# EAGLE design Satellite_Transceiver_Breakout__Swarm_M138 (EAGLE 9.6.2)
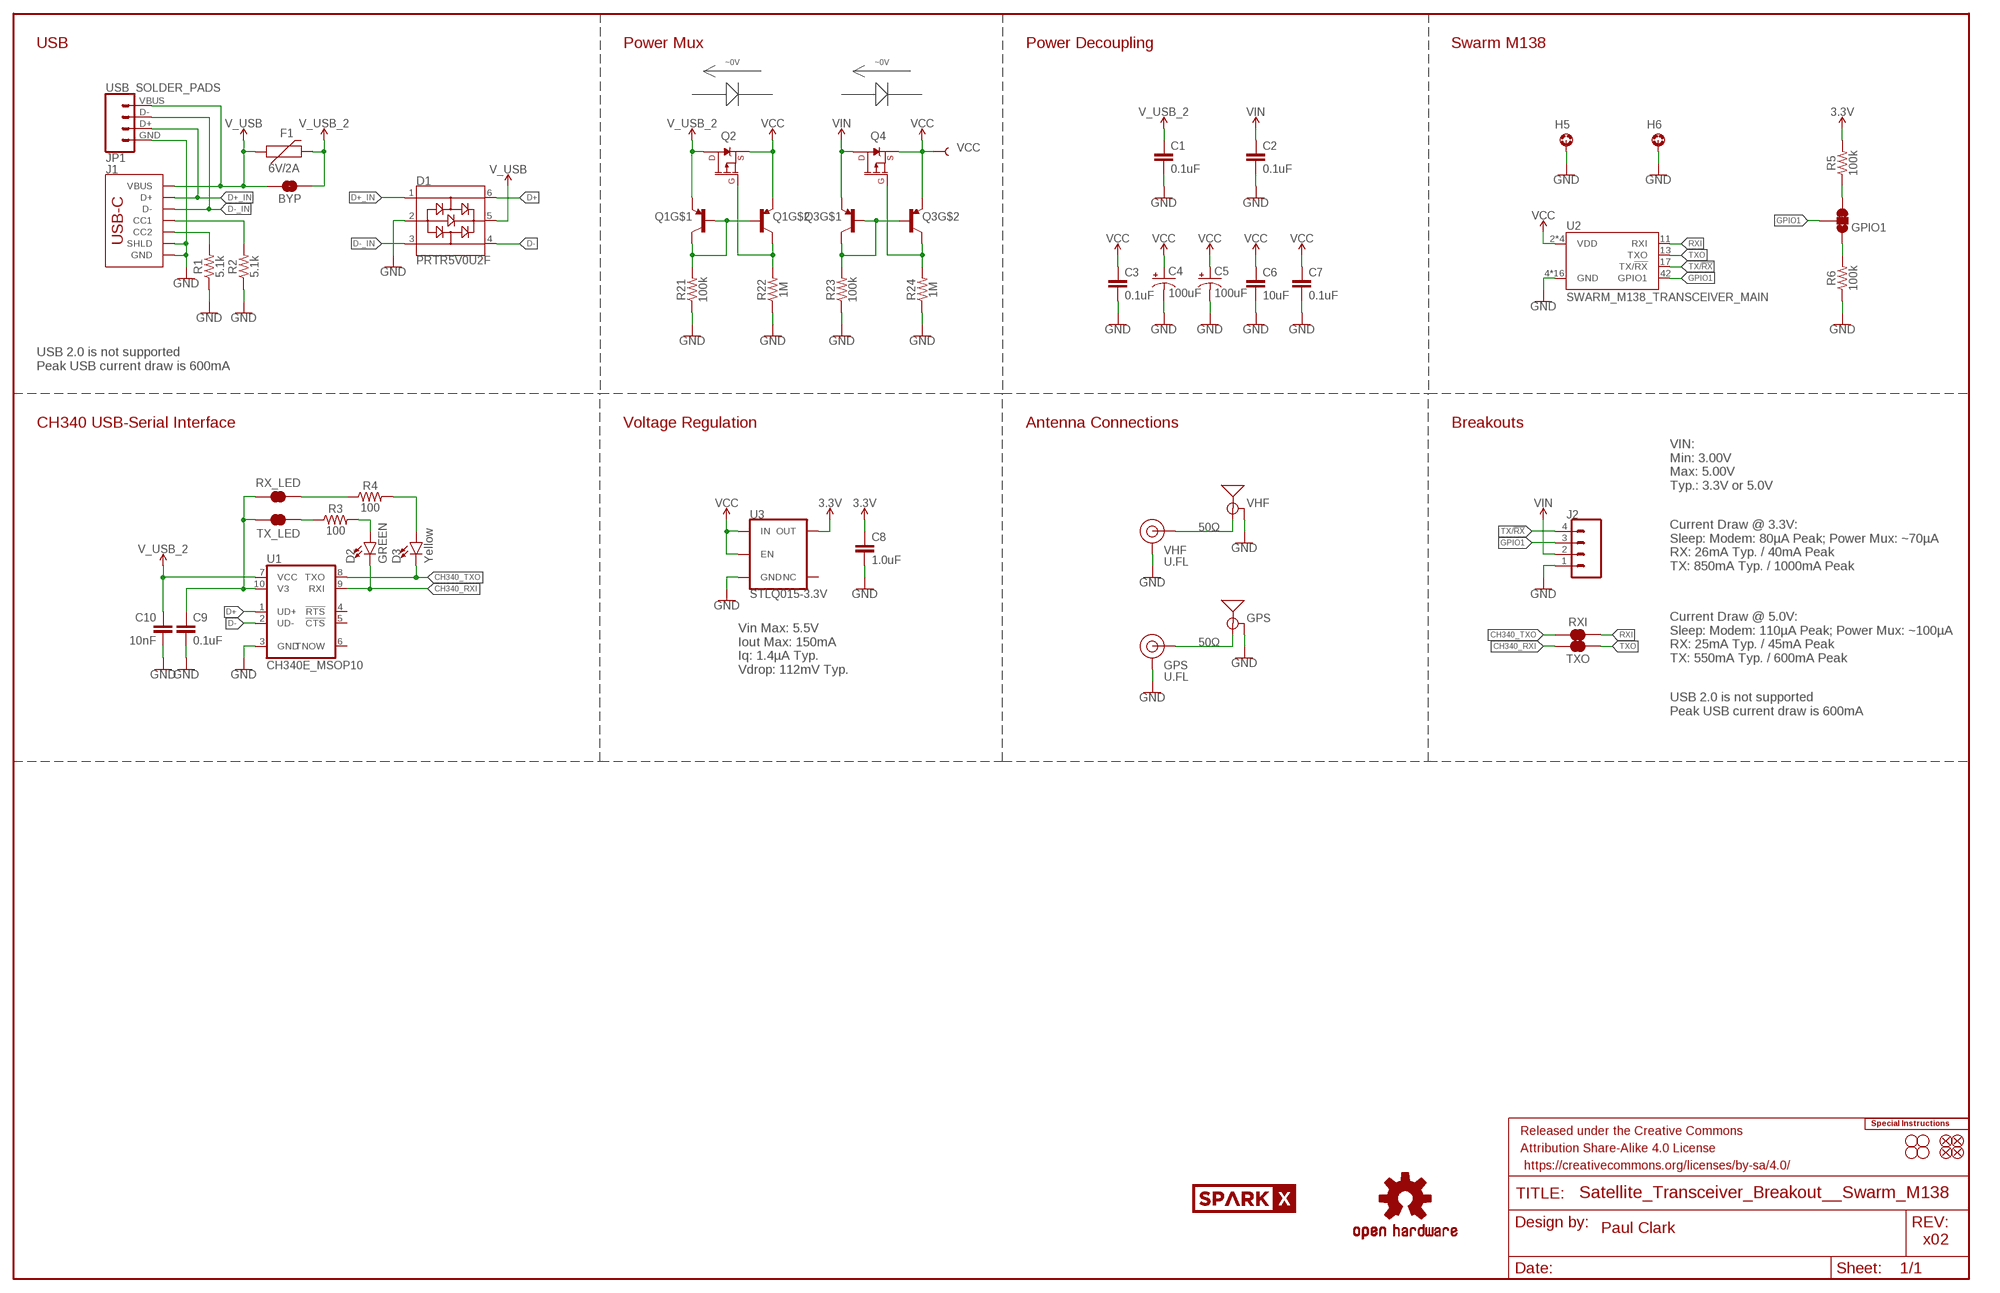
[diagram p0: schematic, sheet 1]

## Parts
BYP  JUMPER-SMT_2_NO_SILK  [SMT-JUMPER_2_NO_SILK]
C1  0.1uF  0.1UF-0603-25V-5%  [0603]
C2  0.1uF  0.1UF-0603-25V-5%  [0603]
C3  0.1uF  0.1UF-0603-25V-5%  [0603]
C4  100uF  100UF-POLAR-25V-20%(ELEC)  [PANASONIC_D]
C5  100uF  100UF-POLAR-25V-20%(ELEC)  [PANASONIC_D]
C6  10uF  10UF-0603-6.3V-20%  [0603]
C7  0.1uF  0.1UF-0603-25V-5%  [0603]
C8  1.0uF  1.0UF-0603-16V-10%-X7R  [0603]
C9  0.1uF  0.1UF-0603-25V-5%  [0603]
C10  10nF  10NF-0603-50V-10%  [0603]
D1  PRTR5V0U2F  [SOT886]
D2  GREEN  LED-GREEN0603  [LED-0603]
D3  Yellow  LED-YELLOW0603  [LED-0603]
E1  VHF  ANTENNA-SMA-GROUNDEDEDGE_SMA  [SMA-EDGE]
E2  GPS  ANTENNA-SMA-GROUNDEDEDGE_SMA  [SMA-EDGE]
F1  6V/2A  PPTC_6V2A  [1210]
FD1  FIDUCIAL1X2  [FIDUCIAL-1X2]
FD2  FIDUCIAL1X2  [FIDUCIAL-1X2]
FD3  FIDUCIAL1X2  [FIDUCIAL-1X2]
FD4  FIDUCIAL1X2  [FIDUCIAL-1X2]
FRAME1  FRAME-LEDGER  [CREATIVE_COMMONS]
GPIO1  JUMPER-SMT_3_1-NC_TRACE_SILK  [SMT-JUMPER_3_1-NC_TRACE_SILK]
GPS  U.FL  U.FL2PIN  [U.FL]
H1  STAND-OFF  [STAND-OFF]
H2  STAND-OFF  [STAND-OFF]
H3  STAND-OFF  [STAND-OFF]
H4  STAND-OFF  [STAND-OFF]
H5  STAND-OFF-REFLOW-M2.5_1.5MM_TALL  [STAND-OFF-REFLOW-M2.5]
H6  STAND-OFF-REFLOW-M2.5_1.5MM_TALL  [STAND-OFF-REFLOW-M2.5]
J1  USB_C_2-LAYER_PADS  [USB-C-16P-2LAYER-PADS]
J2  CONN_041X04_NO_SILK  [1X04_NO_SILK]
JP1  USB_SOLDER_PADS  [USB-SOLDER-PADS]
LOGO1  SPECIAL_INSTRUCTIONS-ORDERING  [ORDERING_INSTRUCTIONS]
LOGO2  OSHW-LOGOM  [OSHW-LOGO-M]
LOGO3  OSHW-LOGOM  [OSHW-LOGO-M]
Q1  TRANS_PNP_DUALSOT-363  [SOT363_PHILIPS]
Q2  20V/4.2A/52mΩ/1.4W  MOSFET_PCH-DMG2305UX-7  [SOT23-3]
Q3  TRANS_PNP_DUALSOT-363  [SOT363_PHILIPS]
Q4  20V/4.2A/52mΩ/1.4W  MOSFET_PCH-DMG2305UX-7  [SOT23-3]
R1  5.1k  5.1KOHM5.1KOHM-0603-1/10W-1%  [0603]
R2  5.1k  5.1KOHM5.1KOHM-0603-1/10W-1%  [0603]
R3  100  100OHM-0603-1/10W-1%  [0603]
R4  100  100OHM-0603-1/10W-1%  [0603]
R5  100k  100KOHM-0603-1/10W-1%  [0603]
R6  100k  100KOHM-0603-1/10W-1%  [0603]
R21  100k  100KOHM-0603-1/10W-1%  [0603]
R22  1M  1MOHM-0603-1/4W-5%  [0603]
R23  100k  100KOHM-0603-1/10W-1%  [0603]
R24  1M  1MOHM-0603-1/4W-5%  [0603]
RX_LED  JUMPER-SMT_2_NC_TRACE_SILK  [SMT-JUMPER_2_NC_TRACE_SILK]
RXI  JUMPER-COMBO_2_NC_TRACE  [COMBO-JUMPER_2_NC_TRACE]
TX_LED  JUMPER-SMT_2_NC_TRACE_SILK  [SMT-JUMPER_2_NC_TRACE_SILK]
TXO  JUMPER-COMBO_2_NC_TRACE  [COMBO-JUMPER_2_NC_TRACE]
U1  CH340E_MSOP10  [MSOP10]
U2  SWARM_M138_TRANSCEIVER_MAIN  [M.2-SWARM-M138-A]
U3  STLQ015-3.3V  [SOT23-5]
U$1  SPARKX-LOGO5  [SPARKX-LARGE]
U$2  SPARKX-LOGO5  [SPARKX-LARGE]
VCC  TEST-POINT3X5  [PAD.03X.05]
VHF  U.FL  U.FL2PIN  [U.FL]

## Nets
3.3V: C8.1 R5.2 U3.5(OUT)
CH340_RXI: D2.C TXO.2 TXO.4 U1.9(RXI)
CH340_TXO: D3.C RXI.1 RXI.3 U1.8(TXO)
D+: D1.6 U1.1(UD+)
D+_IN: D1.1 J1.A6(D+) J1.B6(D+) JP1.D+
D-: D1.4 U1.2(UD-)
D-_IN: D1.3 J1.A7(D-) J1.B7(D-) JP1.D-
GND: C1.2 C2.2 C3.2 C4.- C5.- C6.2 C7.2 C8.2 C9.2 C10.2 D1.2 E1.GND@0(GND) E1.GND@1(GND) E1.GND@2(GND) E1.GND@3(GND) E2.GND@0(GND) E2.GND@1(GND) E2.GND@2(GND) E2.GND@3(GND) GPS.1(GND) GPS.2(GND) H5.1 H6.1 J1.GND J1.GND2(GND) J1.SHLD1(SHLD) J1.SHLD2(SHLD) J1.SHLD3(SHLD) J1.SHLD4(SHLD) J2.1 JP1.GND R1.1 R2.1 R6.1 R21.1 R22.1 R23.1 R24.1 U1.3(GND) U2.4(GND) U2.9(GND) U2.15(GND) U2.18(GND) U2.21(GND) U2.26(GND) U2.27(GND) U2.29(GND) U2.34(GND) U2.35(GND) U2.37(GND) U2.40(GND) U2.43(GND) U2.50(GND) U2.A1(GND) U2.A2(GND) U3.2(GND) VHF.1(GND) VHF.2(GND)
GPIO1: GPIO1.2 J2.3 U2.42(GPIO1)
GPS: E2.SIG(SIGNAL) GPS.FEED(SIGNAL)
N$2: J1.B5(CC2) R1.2
N$3: J1.A5(CC1) R2.2
N$5: Q1.2(B) Q1.5(B) Q1.6(C) R21.2
N$6: C9.1 RX_LED.1 TX_LED.2 U1.10(V3)
N$7: R4.1 RX_LED.2
N$9: D2.A R3.2
N$10: D3.A R4.2
N$12: R3.1 TX_LED.1
N$13: Q1.3(C) Q2.1(G) R22.2
N$14: GPIO1.3 R5.1
N$15: Q3.2(B) Q3.5(B) Q3.6(C) R23.2
N$16: GPIO1.1 R6.2
N$28: Q3.3(C) Q4.1(G) R24.2
RXI: RXI.2 RXI.4 U2.11(RXI)
TX/!RX!: J2.4 U2.17(TX/!RX!)
TXO: TXO.1 TXO.3 U2.13(TXO)
V_USB: BYP.2 D1.5 F1.1 J1.VBUS1(VBUS) J1.VBUS2(VBUS) JP1.VBUS
V_USB_2: BYP.1 C1.1 C10.1 F1.2 Q1.1(E) Q2.3(D) U1.7(VCC)
VCC: C3.1 C4.+ C5.+ C6.1 C7.1 Q1.4(E) Q2.2(S) Q3.4(E) Q4.2(S) U2.2(VDD) U2.39(VDD) U2.41(VDD) U2.52(VDD) U3.1(IN) U3.3(EN) VCC.1
VHF: E1.SIG(SIGNAL) VHF.FEED(SIGNAL)
VIN: C2.1 J2.2 Q3.1(E) Q4.3(D)
Unconnected: U1.4(!RTS) U1.5(!CTS) U1.6(TNOW) U3.4(NC)

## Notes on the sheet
- USB | Power Mux | Power Decoupling | Swarm M138
- ~0V | ~0V
- USB 2.0 is not supported
  Peak USB current draw is 600mA
- CH340 USB-Serial Interface | Voltage Regulation | Antenna Connections | Breakouts
- VIN:
  Min: 3.00V
  Max: 5.00V
  Typ.: 3.3V or 5.0V
- Current Draw @ 3.3V:
  Sleep: Modem: 80µA Peak; Power Mux: ~70µA
  RX: 26mA Typ. / 40mA Peak
  TX: 850mA Typ. / 1000mA Peak
- 50Ω
- Current Draw @ 5.0V:
  Sleep: Modem: 110µA Peak; Power Mux: ~100µA
  RX: 25mA Typ. / 45mA Peak
  TX: 550mA Typ. / 600mA Peak
- Vin Max: 5.5V
  Iout Max: 150mA
  Iq: 1.4µA Typ.
  Vdrop: 112mV Typ.
- 50Ω
- USB 2.0 is not supported
  Peak USB current draw is 600mA
- Paul Clark
- x02

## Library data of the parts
BYP = SparkFun-Jumpers:JUMPER-SMT_2_NO: Normally open jumper
C1-C3 C7 C9 = SparkFun-Capacitors:0.1UF: 0.1µF ceramic capacitors; PROD_ID: CAP-08604
C4 C5 = SparkFun-Capacitors:100UF-POLAR: 100µF polarized capacitors; PROD_ID: CAP-12547
C6 = SparkFun-Capacitors:10UF: 10.0µF ceramic capacitors; PROD_ID: CAP-11015
C8 = SparkFun-Capacitors:1.0UF: 1µF ceramic capacitors; PROD_ID: CAP-13930
C10 = SparkFun-Capacitors:10NF: 0.01uF/10nF/10,000pF ceramic capacitors; PROD_ID: CAP-00867
D1 = SparkFun-IC-Power:PRTR5V0U2: A small ESD protection device. Most commonly used on USB D+/D- signals to protect large, expensive, or especially sensitive USB enabled devices.; PROD_ID: DIO-14084
D2 = SparkFun-LED:LED-GREEN: Green SMD LED; PROD_ID: DIO-00821
D3 = SparkFun-LED:LED-YELLOW: Yellow SMD LED; PROD_ID: DIO-09003
E1 E2 = SparkFun-RF:ANTENNA-SMA-GROUNDED: SMA Antenna Connector w/ Ground; PROD_ID: CONN-08289
F1 = SparkFun-Fuses:PPTC: Resettable Fuse PPTC; PROD_ID: RES-14313
FD1-FD4 = SparkFun-Aesthetics:FIDUCIAL: Fiducial Alignment Points
FRAME1 = SparkFun-Aesthetics:FRAME-LEDGER: Schematic Frame - Ledger
GPIO1 = SparkFun-Jumpers:JUMPER-SMT_3_1-NC_TRACE: Normally closed trace jumper (1 of 2 connections) This jumper has a trace between two pads so it's normally closed (NC). The other connection is normally open (NO). Use a razor knife to open the connection. For best results follow the IPC guidelines for cutting traces: Cutout at least 0.063 mm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
GPS VHF = SparkFun-Connectors:U.FL2PIN: SMD Antenna Connector - U.FL; PROD_ID: CONN-09193; SF_ID: WRL-09144
H1-H4 = SparkFun-Hardware:STAND-OFF: Stand Off
H5 H6 = SparkFun-Hardware:STAND-OFF-REFLOW: Stand Off Reflow Compatible; PROD_ID: HW-16629
J1 = SparkFun-Connectors:USB_C: USB Type C 16Pin Connector Super Speed pins not available on the 16-pin purely SMD connector so this part is best for USB 2.0 implementations. D1 and D2 are tied together enabling D+/- no matter which way the cable is plugged into the connector. The two channel configuration pins (CC1/2) are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; PROD_ID: CONN-14122
J2 = SparkFun-Connectors:CONN_04: Multi connection point. Often used as Generic Header-pin footprint for 0.1 inch spaced/style header connections On any of the 0.1 inch spaced packages, you can populate with these: Break Away Headers - Straight (PRT-00116) Break Away Male Headers - Right Angle (PRT-00553) Female Headers (PRT-00115)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; PROD_ID: CONN-09696
JP1 = SparkFun-Connectors:USB_SOLDER_PADS: Solder pad access to USB pins. Helpful to expose on PCBs so user can attach external USB connector if necessary.
LOGO1 = SparkFun-Aesthetics:SPECIAL_INSTRUCTIONS: Special Ordering/Production Instructions Alert
LOGO2 LOGO3 = SparkFun-Aesthetics:OSHW-LOGO: Open-Source Hardware (OSHW) Logo
Q1 Q3 = SparkFun-DiscreteSemi:TRANS_PNP_DUAL: Dual PNP Transistors in Single Package The BCM857BS puts two PNP transistors in a single package. Bipolar (BJT) Transistor Array 2 PNP (Dual) 45V 100mA 100MHz 200mW Surface Mount SOT-363 Datasheet SparkFun Products: SparkFun Pi Servo HAT V2; PROD_ID: TRANS-14386
Q2 Q4 = SparkFun-DiscreteSemi:MOSFET_PCH: P-channel MOSFETs Voltage controlled devices that allow control of high current outputs. SparkFun Products: SparkFun ESP32 Thing SparkFun ESP8266 Thing SparkFun Pi Servo HAT V2 DMG2305UX-7 (20V/4.2A/SOT23-3); PROD_ID: TRANS-14388
R1 R2 = SparkFun-Resistors:5.1KOHM; PROD_ID: RES-12083
R3 R4 = SparkFun-Resistors:100OHM: 100Ω resistor; PROD_ID: RES-07863
R5 R6 R21 R23 = SparkFun-Resistors:100KOHM: 100kΩ resistor; PROD_ID: RES-07828
R22 R24 = SparkFun-Resistors:1MOHM: 1MΩ resistor; PROD_ID: RES-07868
RX_LED TX_LED = SparkFun-Jumpers:JUMPER-SMT_2_NC_TRACE: Normally closed trace jumper
RXI TXO = SparkFun-Jumpers:JUMPER-COMBO_2_NC_TRACE
U1 = SparkFun-IC-Comms:CH340E; PROD_ID: IC-14135
U2 = Swarm:SWARM_M138_TRANSCEIVER: Swarm M138 Modem Description: A satellite transceiver based on the mPCIe standard.; PROD_ID: CONN-16558
U3 = SparkFun-IC-Power:STLQ015: STLQ015 - 150mA CMOS LDO Regulator w/ Enable 1.4uA quiescent; PROD_ID: IC-15779
U$1 U$2 = SparkX:SPARKX-LOGO
VCC = SparkFun-Connectors:TEST-POINT: SparkFun Test Points

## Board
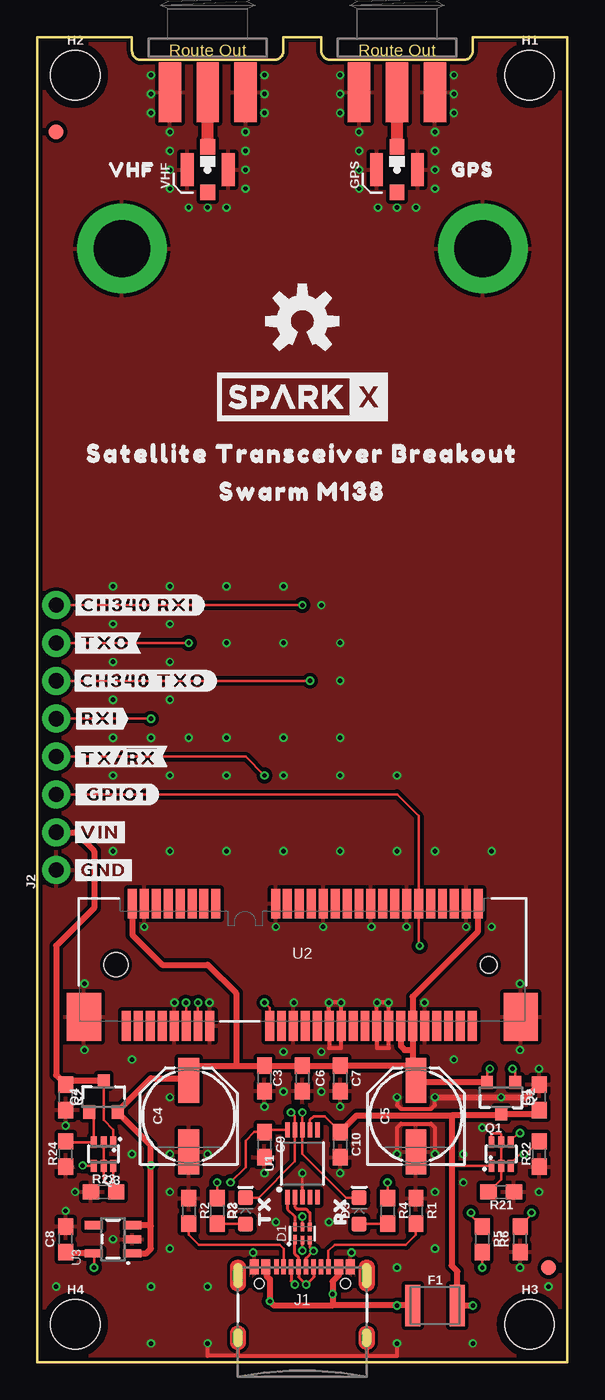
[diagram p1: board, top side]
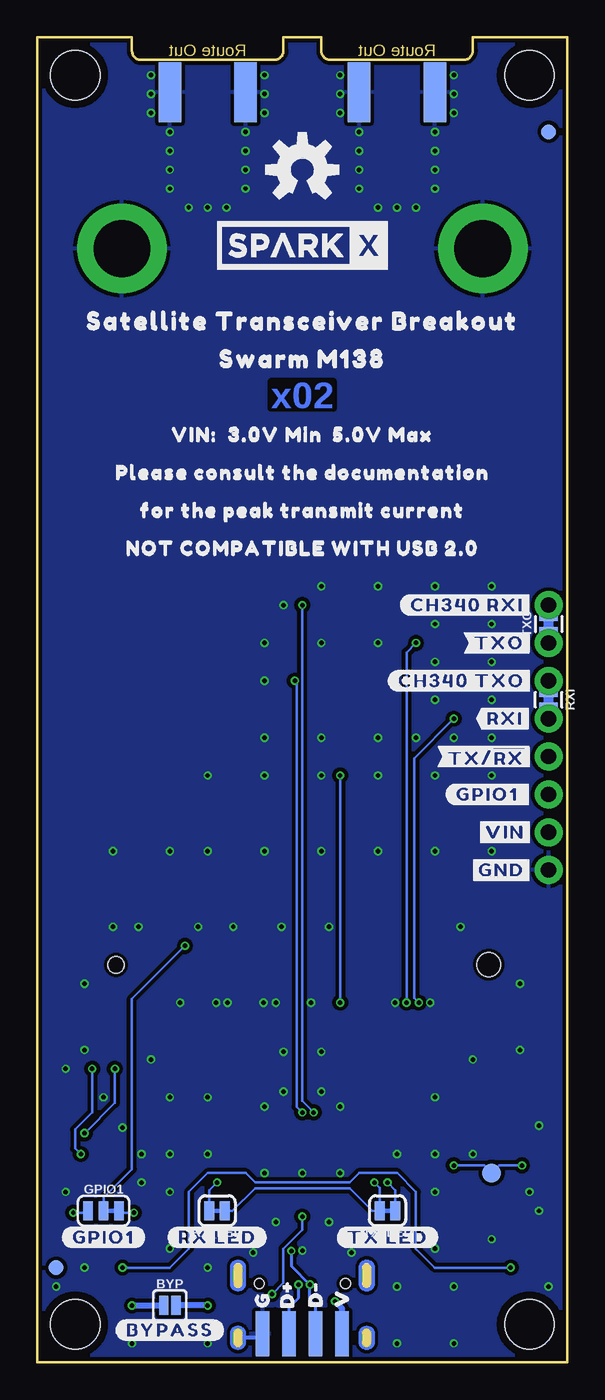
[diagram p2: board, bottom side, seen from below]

Size 35.56 x 88.9 mm. Coordinates in mm from the lower left corner, seen from the top.
Outline: 0,0 35.56,0 35.56,88.9 29.21,88.9 29.21,88.01 arc-90 28.57,87.38 19.68,87.38 arc-90 19.05,88.01 19.05,88.9 16.51,88.9 16.51,88.01 arc-90 15.88,87.38 6.99,87.38 arc-90 6.35,88.01 6.35,88.9 0,88.9 0,0
Copper layers (1*16): Top 0.035mm / dielectric 1.5mm / Bottom 0.035mm
Design rules "SparkFun-2-Layer-Minimum-JLCPCB": minimum track width 5mil, minimum drill 0.3mm, track to track 5mil, track to pad 5mil, pad to pad 5mil, via to via 5mil, smd to smd 5mil, copper to edge 7mil, drill to drill 7mil, minimum pad ring 5mil, minimum via ring 5mil, stop-mask expansion 2.5mil, vias tented up to drill 25mil, thermal gap 10mil
tRestrict: area 10.7,79.1 to 12.2,80.9; area 23.4,79.1 to 24.9,80.9; 4 lines
bRestrict: 3 lines

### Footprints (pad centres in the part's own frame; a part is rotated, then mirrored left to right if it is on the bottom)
SMT-JUMPER_2_NO_SILK = smd 0.635 x 1.27: 1 -0.406,0; 2 0.406,0
0603 = smd 1.1 x 1: 1 -0.85,0; 2 0.85,0
PANASONIC_D = smd 3 x 1.4: + 2.4,0; - -2.4,0
SOT886 = smd 0.61 x 0.25: 1 -0.405,0.5 | smd 0.56 x 0.25: 2 -0.43,0; 3 -0.43,-0.5; 4 0.43,-0.5; 5 0.43,0; 6 0.43,0.5
LED-0603 = smd 1 x 1: A -0.877,0; C 0.877,0
SMA-EDGE = smd 1.5 x 4: GND@0 -2.54,0; GND@1 2.54,0; SIG 0,0 | smd 1.5 x 4 bottom: GND@2 -2.54,0; GND@3 2.54,0
1210 = smd 1 x 2.8: 1 -1.5,0; 2 1.5,0
FIDUCIAL-1X2 = smd 1 x 1: 1 0,0
SMT-JUMPER_3_1-NC_TRACE_SILK = smd 0.66 x 1.27: 1 -1.041,0; 2 0,0; 3 1.041,0
U.FL = smd 2.2 x 0.85: 1 0,1.375; 2 0,-1.375 | smd 1.05 x 1: FEED 1.525,0; NC -1.525,0
STAND-OFF = hole 3.302: 0,0
STAND-OFF-REFLOW-M2.5 = drill 3.8 pad 6: 1 0,0
USB-C-16P-2LAYER-PADS = smd 0.3 x 1: A5 -1.25,-0.34; A6 -0.25,-0.34; A7 0.25,-0.34; A8 1.25,-0.34; B5 1.75,-0.34; B6 0.75,-0.34; B7 -0.75,-0.34; B8 -1.75,-0.34 | smd 0.6 x 1: GND -3.225,-0.34; GND2 3.225,-0.34; VBUS1 -2.45,-0.34; VBUS2 2.45,-0.34 | drill 0.4 pad 0.6 long: SHLD1 -4.318,-0.915; SHLD2 4.318,-0.915; SHLD3 -4.318,-5.095; SHLD4 4.318,-5.095 | hole 0.65: -2.89,-1.445; 2.89,-1.445
1X04_NO_SILK = drill 1.016 pad 1.88: 1 0,0; 2 2.54,0; 3 5.08,0; 4 7.62,0
USB-SOLDER-PADS = smd 3 x 0.9: D+ 0,-0.889; D- 0,0.889; GND 0,-2.667; VBUS 0,2.667
SOT363_PHILIPS = smd 0.4 x 0.8: 1 -0.65,-0.8; 2 0,-0.8; 3 0.65,-0.8; 4 0.65,0.8; 5 0,0.8; 6 -0.65,0.8
SOT23-3 = smd 0.8 x 0.9: 1 -0.95,-1; 2 0.95,-1; 3 0,1.1
SMT-JUMPER_2_NC_TRACE_SILK = smd 0.66 x 1.27: 1 -0.521,0; 2 0.521,0
COMBO-JUMPER_2_NC_TRACE = smd 0.635 x 1.27: 1 -0.508,0; 2 0.508,0 | drill 1.016 pad 1.88: 3 -1.27,0; 4 1.27,0
MSOP10 = smd 1 x 0.3: 1 -2.25,1; 2 -2.25,0.5; 3 -2.25,0; 4 -2.25,-0.5; 5 -2.25,-1; 6 2.25,-1; 7 2.25,-0.5; 8 2.25,0; 9 2.25,0.5; 10 2.25,1
M.2-SWARM-M138-A = smd 0.6 x 2: 1 -11.8,-4.1; 2 -11.4,4.1; 3 -11,-4.1; 4 -10.6,4.1; 5 -10.2,-4.1; 6 -9.8,4.1; 7 -9.4,-4.1; 8 -9,4.1; 9 -8.6,-4.1; 10 -8.2,4.1; 11 -7.8,-4.1; 12 -7.4,4.1; 13 -7,-4.1; 14 -6.6,4.1; 15 -6.2,-4.1; 16 -5.8,4.1; 17 -2.2,-4.1; 18 -1.8,4.1; 19 -1.4,-4.1; 20 -1,4.1; 21 -0.6,-4.1; 22 -0.2,4.1; 23 0.2,-4.1; 24 0.6,4.1; 25 1,-4.1; 26 1.4,4.1; 27 1.8,-4.1; 28 2.2,4.1; 29 2.6,-4.1; 30 3,4.1; 31 3.4,-4.1; 32 3.8,4.1; 33 4.2,-4.1; 34 4.6,4.1; 35 5,-4.1; 36 5.4,4.1; 37 5.8,-4.1; 38 6.2,4.1; 39 6.6,-4.1; 40 7,4.1; 41 7.4,-4.1; 42 7.8,4.1; 43 8.2,-4.1; 44 8.6,4.1; 45 9,-4.1; 46 9.4,4.1; 47 9.8,-4.1; 48 10.2,4.1; 49 10.6,-4.1; 50 11,4.1; 51 11.4,-4.1; 52 11.8,4.1 | smd 2.3 x 3.2: A1 -14.65,-3.5; A2 14.65,-3.5 | hole 1.1: 12.5,0 | hole 1.6: -12.5,0
SOT23-5 = smd 0.55 x 1.2: 1 -0.95,-1.3; 2 0,-1.3; 3 0.95,-1.3; 4 0.95,1.3; 5 -0.95,1.3
PAD.03X.05 = smd 1.27 x 1.27: 1 0,0

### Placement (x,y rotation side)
BYP  26.67,3.81 0 bottom
C1  33.66,17.78 90 top
C2  1.91,17.78 270 top
C3  15.24,19.05 270 top
C4  10.16,16.51 90 top
C5  25.4,16.51 90 top
C6  17.78,19.05 270 top
C7  20.32,19.05 270 top
C8  1.91,8.26 90 top
C9  15.24,14.61 270 top
C10  20.32,14.61 270 top
D1  17.78,8.64 90 top
D2  13.97,10.16 90 top
D3  21.59,10.16 90 top
E1  11.43,85.22 0 top
E2  24.13,85.22 0 top
F1  26.67,3.81 0 top
FD1  34.29,6.35 0 top
FD2  34.29,6.35 0 bottom
FD3  1.27,82.55 0 top
FD4  1.27,82.55 0 bottom
FRAME1  not placed on the board
GPIO1  31.11,10.16 0 bottom
GPS  24.13,80.01 90 top
H1  33.02,86.36 0 top
H2  2.54,86.36 0 top
H3  33.02,2.54 0 top
H4  2.54,2.54 0 top
H5  5.68,74.72 0 top
H6  29.88,74.72 0 top
J1  17.78,6.73 0 top
J2  1.27,33.02 90 top
JP1  17.78,1.91 270 bottom
LOGO1  not placed on the board
LOGO2  17.78,69.85 0 top
LOGO3  17.78,80.01 0 bottom
Q1  31.11,13.97 0 top
Q2  31.11,17.78 180 top
Q3  4.45,13.97 180 top
Q4  4.45,17.78 0 top
R1  25.4,10.16 270 top
R2  10.16,10.16 270 top
R3  12.06,10.16 270 top
R4  23.5,10.16 270 top
R5  29.84,8.26 270 top
R6  32.38,8.26 90 top
R21  31.11,11.43 180 top
R22  33.66,13.97 90 top
R23  4.45,11.43 0 top
R24  1.91,13.97 90 top
RX_LED  23.5,10.16 180 bottom
RXI  1.27,44.45 270 bottom
TX_LED  12.06,10.16 180 bottom
TXO  1.27,49.53 90 bottom
U1  17.78,13.34 90 top
U2  17.78,26.67 0 top
U3  5.08,8.26 90 top
U$1  17.78,74.93 0 bottom
U$2  17.78,64.77 0 top
U$3  [VHF0]  6.35,80.01 0 top
U$4  [GPS0]  29.21,80.01 0 top
U$5  [VIN#__3#0V_MIN__5#0V_MAX0]  17.78,62.23 0 bottom
U$6  [PLEASE_CONSULT_THE_DOCUMENTATION0]  17.78,59.69 0 bottom
U$7  [#CH340_RXI#0]  6.73,50.8 0 top
U$8  [#CH340_RXI#341]  6.73,50.8 0 bottom
U$9  [#TXO#341]  4.57,48.26 0 top
U$10  [#TXO#342]  4.57,48.26 0 bottom
U$11  [#CH340_TXO#0]  7.11,45.72 0 top
U$12  [#CH340_TXO#341]  7.11,45.72 0 bottom
U$13  [#RXI#0]  4.19,43.18 0 bottom
U$14  [#RXI#1]  4.19,43.18 0 top
U$15  [#TX##RX##1]  5.46,40.64 0 bottom
U$16  [#TX##RX##0]  5.46,40.64 0 top
U$17  [#GPIO1_#2]  5.21,38.1 0 bottom
U$18  [V0]  15.11,4.32 90 bottom
U$19  [#GPIO1#0]  31.11,8.38 0 bottom
U$20  [#_GPIO1#2]  5.21,38.1 0 top
U$21  [#VIN#0]  4.19,35.56 0 top
U$22  [#VIN#0]  4.19,35.56 0 bottom
U$23  [#GND#0]  4.45,33.02 0 top
U$24  [#GND#0]  4.45,33.02 0 bottom
U$25  [TX0]  15.24,10.16 90 top
U$26  [RX0]  20.32,10.16 90 top
U$27  [#TX_LED#0]  12.06,8.38 0 bottom
U$28  [#RX_LED#0]  23.5,8.38 0 bottom
U$29  [#BYPASS#0]  26.67,2.16 0 bottom
U$30  [G3]  20.45,4.19 90 bottom
U$31  [FOR_THE_PEAK_TRANSMIT_CURRENT1]  17.78,57.15 0 bottom
U$32  [NOT_COMPATIBLE_WITH_USB_2#02]  17.78,54.61 0 bottom
U$34  [SATELLITE_TRANSCEIVER_BREAKOUT0]  17.78,60.96 0 top
U$36  [D#2]  18.8,4.57 90 bottom
U$37  [D#1]  16.89,4.57 90 bottom
U$39  [SATELLITE_TRANSCEIVER_BREAKOUT0]  17.78,69.85 0 bottom
U$40  [SWARM_M1381]  17.78,58.42 0 top
U$41  [SWARM_M1381]  17.78,67.31 0 bottom
VCC  5.08,12.7 0 bottom
VHF  11.43,80.01 90 top

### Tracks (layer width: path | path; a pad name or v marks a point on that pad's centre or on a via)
3.3V  (via drill 0.3)
  Top 0.152: U3.5 3.81,7.28 v3.81,6.35 | v29.84,6.35 R5.2
  Top 0.406: U3.5 2,7.3 C8.1
  Bottom 0.152: v29.84,6.35 26.67,6.35 25.4,7.62 25.4,11.43 24.13,12.7 21.59,12.7 20.95,12.06 14.61,12.06 13.97,12.7 11.43,12.7 10.16,11.43 10.16,7.62 8.89,6.35 v3.81,6.35
CH340_RXI  (via drill 0.3)
  Top 0.152: D2.C 14.85,11.04 17.28,13.47 U1.9 17.28,16.5 v17.02,16.76 | TXO.4 v17.78,50.8
  Bottom 0.152: TXO.4 TXO.2 | v17.02,16.76 17.78,17.53 v17.78,50.8
CH340_TXO  (via drill 0.3)
  Top 0.152: D3.C 20.71,11.04 17.78,13.97 U1.8 v17.78,16.76 | v18.29,45.72 RXI.3
  Bottom 0.152: RXI.3 RXI.1 | v17.78,16.76 18.16,17.14 18.16,45.59 v18.29,45.72
D+
  Top 0.203: U1.1 16.78,10.27 17.27,9.78 D1.6
D+_IN  (via drill 0.3)
  Top 0.203: D1.1 17.27,7.29 17.53,7.03 J1.A6 17.53,5.71 v18.03,5.21 18.53,5.7 J1.B6
  Bottom 0.203: v18.03,5.21 18.03,4.32 18.67,3.68 JP1.D+
D-
  Top 0.203: U1.2 17.28,10.41 17.4,10.29 18.03,10.29 18.29,10.03 D1.4
D-_IN  (via drill 0.3)
  Top 0.203: J1.A7 18.03,6.98 v18.52,7.47 18.28,7.71 D1.3 | J1.B7 17.03,5.45 v17.27,5.21
  Bottom 0.203: v18.52,7.47 18.52,6.46 v17.27,5.21 17.27,4.19 16.89,3.81 JP1.D-
GND  (via drill 0.3)
  Top 0.152: v17.78,7.49 D1.2 | U1.3 v17.78,12.7
  Top 0.254: v24.13,17.78 24.13,17.26 24.38,17.01 26.42,17.01 26.67,17.26 v26.67,17.78 | v24.13,13.97 24.13,15.75 24.38,16 26.42,16 26.67,15.75 v26.67,13.97 | J1.SHLD3 13.46,0.43 | 13.46,0.43 11.43,0.43 v11.43,1.27 | J1.SHLD4 22.1,0.43 | 22.1,0.43 24.13,0.43 v24.13,1.27 | 13.46,0.43 22.1,0.43 | U2.27 19.56,22.57 v19.56,24.13 v20.38,24.13 U2.29 20.38,21.08 19.58,21.08 U2.27 | U2.35 22.78,24.13 v22.8,24.13 v23.56,24.13 23.58,24.13 U2.37 23.58,21.08 22.78,21.08 U2.35
  Top 0.406: v26.67,17.78 32.8,17.78 C1.2
  Bottom 0.254: JP1.GND 20.72,1.64 J1.SHLD4
  other vias: 7.62,86.36 7.62,83.82 8.89,82.55 8.89,81.28 8.89,78.74 10.16,77.47 12.7,77.47 13.97,78.74 13.97,81.28 13.97,82.55 15.24,83.82 15.24,86.36 20.32,86.36 20.32,83.82 21.59,82.55 21.59,81.28 21.59,78.74 22.86,77.47 25.4,77.47 26.67,78.74 26.67,81.28 26.67,82.55 27.94,83.82 27.94,86.36 7.62,85.09 8.89,80.01 15.24,85.09 13.97,80.01 11.43,77.47 20.32,85.09 27.94,85.09 26.67,80.01 21.59,80.01 24.13,77.47 7.18,29.21 16,29.21 19.18,29.21 22.42,29.21 24.77,29.21 9.21,24.13 17.21,24.13 11.56,24.13 28.77,29.21 25.97,24.13 32.38,25.4 32.38,20.95 3.17,25.4 3.17,20.95 8.89,13.97 11.43,13.97 15.24,12.7 20.32,12.7 15.24,17.14 19.05,18.16 20.32,17.14 2.54,11.43 1.91,10.16 5.08,8.26 7.62,5.08 14.48,7.37 21.08,7.37 33.66,11.43 32.38,6.35 16.51,18.16 11.43,5.08 29.21,1.27 7.62,1.27 1.27,5.08 34.29,5.08 26.67,11.43 8.89,11.43 16,9.4 19.56,9.4 8.89,17.78 33.66,19.68 31.11,17.78 27.94,20.32 6.35,20.32 5.08,34.29 8.89,34.29 12.7,34.29 16.51,34.29 20.32,34.29 24.13,34.29 26.67,34.29 8.89,39.37 5.08,39.37 12.7,39.37 16.51,39.37 20.32,39.37 24.13,39.37 5.08,41.91 12.7,41.91 16.51,41.91 20.32,41.91 5.08,44.45 8.89,44.45 20.32,45.72 20.32,48.26 16.51,48.26 12.7,48.26 8.89,46.99 5.08,46.99 5.08,49.53 8.89,49.53 5.08,52.07 8.89,52.07 12.7,52.07 16.51,52.07 19.05,50.8 1.91,15.88 29.84,15.75 28.57,12.06 30.48,34.29 30.48,29.21 28.57,13.97 24.13,6.35 26.67,7.62 8.89,7.62 19.05,20.83 16.51,20.83 6.35,13.97 7.62,41.91 10.16,41.91
  pour Top (isolate 0.254): 0,0 0,88.9 35.56,88.9 35.56,0
  pour Bottom (isolate 0.254): 0,0 0,88.9 35.56,88.9 35.56,0
GPIO1  (via drill 0.3)
  Top 0.152: v25.65,27.94 25.58,28.01 U2.42 25.58,36.65 24.13,38.1 J2.3
  Bottom 0.152: GPIO1.2 31.11,11.05 29.21,12.95 29.21,24.38 v25.65,27.94
GPS
  Top 0.813: GPS.FEED E2.SIG
N$2
  Top 0.152: R1.2 25.4,8.55 24.73,7.87 19.94,7.87 19.53,7.46 J1.B5
N$3
  Top 0.152: R2.2 10.16,8.55 10.83,7.87 16.26,7.87 16.53,7.6 J1.A5
N$5
  Top 0.152: R21.2 31.11,12.28 Q1.2 Q1.5 31.11,15.3 31.05,15.37 30.54,15.37 30.46,15.29 Q1.6
N$6  (via drill 0.3)
  Top 0.152: U1.10 15.37,15.59 C9.1 14.57,15.46 13.97,14.86 13.97,13.08 v12.95,12.06
  Bottom 0.152: RX_LED.1 22.48,10.16 20.95,11.68 14.61,11.68 13.08,10.16 TX_LED.2 12.59,11.7 v12.95,12.06
N$7  (via drill 0.3)
  Top 0.152: R4.1 v23.5,12.06
  Bottom 0.152: v23.5,12.06 24.02,11.54 RX_LED.2
N$9
  Top 0.152: R3.2 12.09,9.28 D2.A
N$10
  Top 0.152: D3.A 23.47,9.28 R4.2
N$12  (via drill 0.3)
  Top 0.152: R3.1 v12.06,12.06
  Bottom 0.152: TX_LED.1 11.54,11.54 v12.06,12.06
N$13  (via drill 0.3)
  Top 0.152: v31.88,19.68 32.06,19.5 Q2.1 | R22.2 32.8,13.97 v32.64,13.97 32.38,13.97 31.77,13.35 Q1.3
  Bottom 0.152: v31.88,19.68 31.88,16.76 33.02,15.62 33.02,14.35 v32.64,13.97
N$14  (via drill 0.3)
  Top 0.152: R5.1 29.08,9.87 v29.08,10.03
  Bottom 0.152: GPIO1.3 29.95,10.03 v29.08,10.03
N$15
  Top 0.152: Q3.2 Q3.5 4.45,12.28 R23.2 5.09,11.63 Q3.6
N$16  (via drill 0.3)
  Top 0.152: v33.15,10.03 33.15,9.91 32.38,9.14 R6.2
  Bottom 0.152: v33.15,10.03 32.28,10.03 GPIO1.1
N$28
  Top 0.152: Q4.1 3.79,16.48 Q3.3 1.96,14.77 R24.2
RXI  (via drill 0.3)
  Top 0.152: U2.11 9.98,24.12 v9.97,24.13 | v7.62,43.18 RXI.4
  Bottom 0.152: v9.97,24.13 10.29,24.45 10.29,40.51 v7.62,43.18 | RXI.4 RXI.2
TX/!RX!  (via drill 0.3)
  Top 0.152: v15.24,39.37 13.97,40.64 J2.4 | v15.24,24.13 15.58,23.79 U2.17
  Bottom 0.152: v15.24,39.37 v15.24,24.13
TXO  (via drill 0.3)
  Top 0.152: U2.13 10.78,24.11 v10.79,24.13 | v10.16,48.26 TXO.3
  Bottom 0.152: v10.79,24.13 10.79,47.62 v10.16,48.26 | TXO.3 TXO.1
V_USB  (via drill 0.3)
  Top 0.152: D1.5 v17.78,9.78
  Top 0.406: J1.VBUS1 15.37,6.35 15.37,5.81 15.6,5.58 v15.6,4.09 15.88,3.81 19.81,3.81 | J1.VBUS2 20.23,5.84 19.81,5.43 v19.81,4.57 19.81,3.81 | F1.1 v24.13,3.81 19.81,3.81
  Bottom 0.152: v17.78,9.78 17.78,8.89 19.05,7.62 19.05,5.33 v19.81,4.57
  Bottom 0.406: v24.13,3.81 BYP.2 | v15.6,4.09 15.11,3.61 JP1.VBUS
V_USB_2  (via drill 0.3)
  Top 0.152: U1.7 18.28,16.25 18.54,16.51 19.27,16.51 C10.1 | Q1.1 27.83,13.17 27.79,13.21
  Top 0.406: v29.21,3.81 F1.2 28.17,6.1 27.79,6.48 27.79,13.21 27.79,16.55 | C1.1 33.41,16.68 Q2.3 30.99,16.55 27.79,16.55 | C10.1 21.42,16.55 27.79,16.55
  Bottom 0.406: v29.21,3.81 BYP.1
VCC  (via drill 0.3)
  Top 0.152: Q3.4 3.09,13.17 v3.05,13.21 | Q2.2 30.16,19.5 v30.35,19.68 | v32.38,15.37 32.26,15.37 31.77,14.87 Q1.4
  Top 0.406: 13.34,19.9 10.5,19.9 10.16,19.56 C4.+ 10.02,19.05 7.62,19.05 5.39,16.82 Q4.2 7.62,14.55 v7.62,13.21 7.62,9.14 | 13.34,19.9 C3.1 C6.1 C7.1 25.31,19.9 25.4,19.81 C5.+ | 25.18,20.95 U2.41 25.18,24.51 29.54,28.87 29.54,30.73 U2.52 | 25.18,20.95 25.18,19.13 C5.+ | U2.2 6.38,28.67 8.38,26.67 11.43,26.67 13.34,24.77 13.34,19.9 | Q2.2 25.53,18.78 C5.+ | U2.39 24.38,21.21 24.64,20.95 25.18,20.95 | U3.1 7.3,7.3 7.62,7.62 7.62,9.14 | U3.3 7.56,9.21 7.62,9.14
  Bottom 0.152: v7.62,13.21 5.59,13.21 VCC.1 4.57,13.21 v3.05,13.21 | v30.35,19.68 30.35,17.4 v32.38,15.37
VHF
  Top 0.813: VHF.FEED E1.SIG
VIN
  Top 0.152: Q4.3 4.45,16.26 5.09,15.61 Q3.1
  Top 0.406: J2.2 2.54,35.56 3.81,34.29 3.81,30.48 1.27,27.94 1.27,19.27 C2.1 2.15,18.88 Q4.3

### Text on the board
Bottom: x02
Milling: Route Out | Route Out
Measures: Dimensions In Inches
tDocu: 2-Layer Board / 1.6mm Thickness / 1oz Copper / Lead-Free HASL Finish | Paul Clark

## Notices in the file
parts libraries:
SparkFun-Aesthetics: Licensing: Creative Commons ShareAlike 4.0 International - https://creativecommons.org/licenses/by-sa/4.0
SparkFun-Aesthetics: Released under the Creative Commons Attribution Share-Alike 4.0 License
SparkFun-Aesthetics: https://creativecommons.org/licenses/by-sa/4.0
